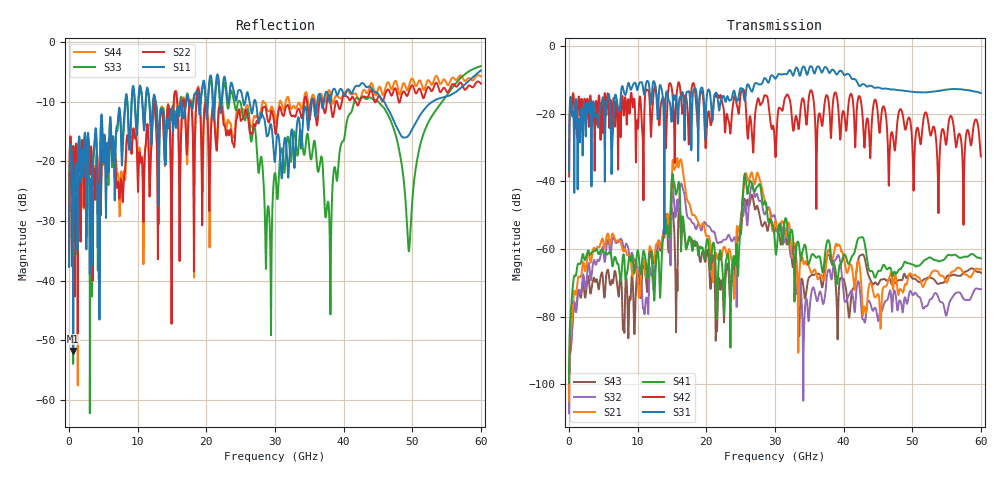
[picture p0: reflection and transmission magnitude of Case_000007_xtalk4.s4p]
! Info: Touchstone file created by circ.  Input file=CasetestDOE_NRZ_template_000007.circ
# Hz S RI R 50
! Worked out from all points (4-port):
!   6000 points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, 10 MHz to 60 GHz, reference 50 ohm
!   strongest paths, dB at 10 MHz, 15.01 GHz, 30.01 GHz, 45.01 GHz, 60 GHz:
!     S31: -37.0, -20.1, -9.6, -12.2, -13.9
!     S42: -38.5, -13.1, -30.5, -20.6, -32.6
!     S41: -99.6, -38.7, -58.8, -66.6, -62.7
!     S21: -104.9, -37.2, -51.8, -73.3, -65.9
!     S32: -108.5, -43.0, -50.5, -81.2, -71.8
!     S43: -106.7, -49.5, -54.3, -70.5, -67.0
!   lowest |S11| = -51.8 dB at 600 MHz (marker M1), VSWR 1.01, Z = 49.9 - j0.224 ohm
!   |S11| at or under -10 dB: start of sweep to 8.188 GHz; 27.19 GHz to 35.26 GHz (8.075 GHz wide, 25.9 % of centre); 45.89 GHz to 52.95 GHz (7.051 GHz wide, 14.3 % of centre)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
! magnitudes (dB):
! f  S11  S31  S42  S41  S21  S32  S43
! 10 MHz  -37.7  -37.0  -38.5  -99.6  -104.9  -108.5  -106.7
! 600 MHz  -51.8  -19.3  -13.9  -69.9  -75.3  -79.0  -78.3
! 16.01 GHz  -12.1  -17.0  -10.7  -40.2  -35.1  -46.6  -46.9
! 23.98 GHz  -8.1  -13.2  -15.9  -62.0  -71.9  -56.9  -63.7
! 26.55 GHz  -11.7  -13.3  -23.2  -40.1  -37.4  -41.4  -44.3
! 34.18 GHz  -12.0  -6.0  -15.9  -59.4  -64.4  -89.4  -71.9
! 60 GHz  -4.8  -13.9  -32.6  -62.7  -65.9  -71.8  -67.0
